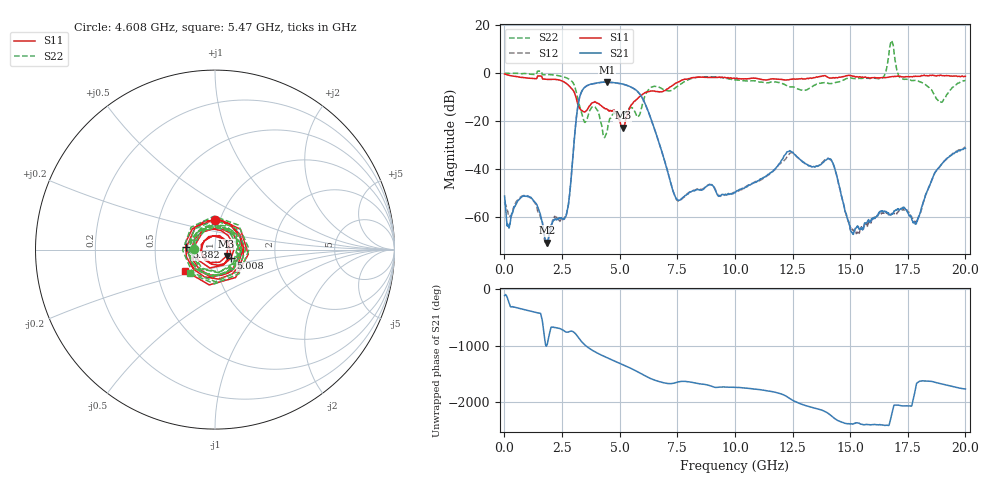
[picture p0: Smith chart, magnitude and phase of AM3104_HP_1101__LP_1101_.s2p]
!Created with skrf (http://scikit-rf.org).
# Hz S RI R 50.0
!freq ReS11 ImS11 ReS21 ImS21 ReS12 ImS12 ReS22 ImS22
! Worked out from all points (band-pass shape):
!   1601 points, 10 MHz to 20 GHz, reference 50 ohm
!   highest |S21| = -3.72 dB at 4.458 GHz (marker M1); lowest = -70.5 dB at 1.859 GHz (marker M2)
!   |S21| within 3 dB of the highest: 3.412 GHz to 5.659 GHz (2.247 GHz wide, 49.5 % of centre)
!   lowest |S11| = -22.7 dB at 5.132 GHz (marker M3), VSWR 1.16, Z = 56.7 - j4.06 ohm
!   |S11| at or under -10 dB: 3.106 GHz to 5.84 GHz (2.734 GHz wide, 61.1 % of centre)
!   |S22| runs from -26.8 to 13.6 dB; largest |S21 - S12| = 0.069
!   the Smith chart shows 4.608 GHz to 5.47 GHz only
!   S11 on the Smith chart (normalised r, x): 4.608 GHz: 0.94, +0.32; 5.008 GHz: 1.19, -0.12; 5.382 GHz: 0.72, +0.02; 5.47 GHz: 0.70, -0.17
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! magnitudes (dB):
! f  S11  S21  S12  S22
! 10 MHz  -0.4  -51.2  -53.6  0.0
! 1.159 GHz  -2.2  -51.8  -52.2  -0.5
! 1.859 GHz  -2.6  -70.5  -71.7  -0.6
! 2.709 GHz  -4.4  -58.1  -58.1  -2.1
! 3.346 GHz  -15.5  -7.8  -7.9  -16.5
! 4.458 GHz  -15.1  -3.7  -3.7  -24.4
! 4.608 GHz  -15.6  -3.8  -3.9  -18.8
! 5.008 GHz  -19.9  -4.3  -4.4  -17.6
! 5.132 GHz  -22.7  -4.6  -4.6  -17.9
! 5.382 GHz  -15.9  -5.3  -5.4  -14.9
! 5.47 GHz  -13.8  -5.7  -5.7  -14.4
! 6.682 GHz  -7.8  -28.1  -28.2  -5.7
! 7.519 GHz  -3.8  -52.8  -53.1  -5.5
! 10.01 GHz  -2.3  -49.8  -49.7  -2.9
! 12.34 GHz  -2.8  -32.6  -33.9  -5.6
! 13.34 GHz  -2.1  -39.0  -38.9  -5.7
! 14.22 GHz  -2.1  -36.9  -37.0  -4.3
! 15.1 GHz  -1.3  -66.5  -65.0  -2.2
! 16.68 GHz  -1.6  -58.6  -58.9  7.2
! 17.84 GHz  -1.3  -62.9  -61.8  -3.1
! 18.93 GHz  -0.8  -38.4  -38.5  -12.1
! 20 GHz  -1.3  -31.3  -30.8  -3.1
